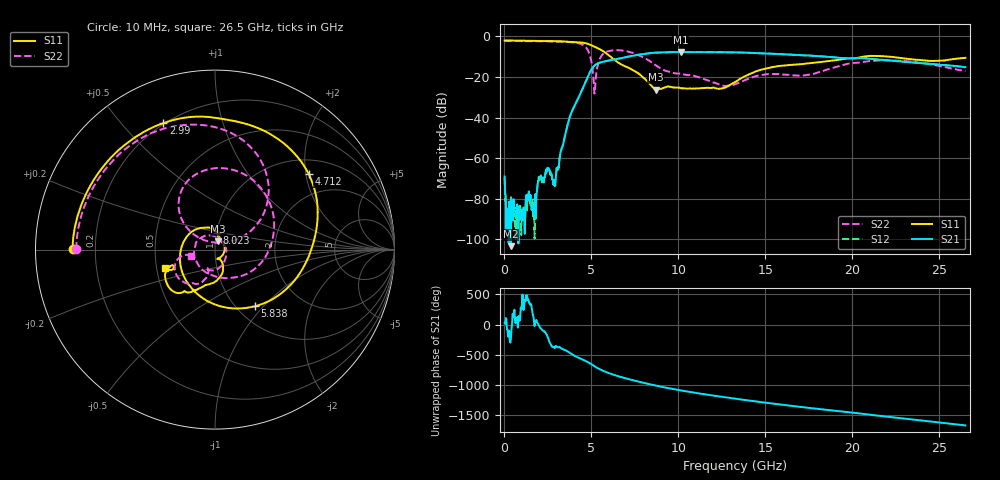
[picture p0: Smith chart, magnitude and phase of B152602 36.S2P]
!  2-Port S-parameters saved by WinCal
! VAR MeasName=S-Parameters (CALIBRATED_DATA) read from VNA (N5242A)
! VAR MeasDate=2016-1-5 16:31:28
! VAR NAME=B152602 36
! VAR FILENAME=B152602 36.S2P
! VAR DATE=2016-1-5 16:31:28
! VAR PHYS_PORTS=1,2
# Hz S DB R 50
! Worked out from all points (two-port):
!   801 points, 10 MHz to 26.5 GHz, reference 50 ohm
!   highest |S21| = -7.67 dB at 10.14 GHz (marker M1); lowest = -103.3 dB at 374.2 MHz (marker M2)
!   |S21| within 3 dB of the highest: 6.748 GHz to 19.42 GHz (12.67 GHz wide, 96.8 % of centre); 20.43028 GHz to 20.45867 GHz (28.39 MHz wide, 0.139 % of centre)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
!   lowest |S11| = -26.2 dB at 8.685 GHz (marker M3), VSWR 1.10, Z = 51.6 + j4.71 ohm
!   |S11| at or under -10 dB: 6.094 GHz to 20.61 GHz (14.51 GHz wide, 109 % of centre); 22.15 GHz to end of sweep
!   |S22| runs from -28.1 to -2.2 dB; largest |S21 - S12| = 0.0032
!   S11 on the Smith chart (normalised r, x): 10 MHz: 0.12, +0.00; 2.99 GHz: 0.20, +0.65; 4.712 GHz: 1.35, +2.07; 5.838 GHz: 1.21, -0.90; 8.023 GHz: 1.01, +0.19; 26.5 GHz: 0.55, -0.12
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1e7  -2.01 179.7  -68.96 24.1  -69.51 1.8  -2.24 179.8
3.742375e8  -2.04 172.2  -103.30 139.0  -79.12 179.1  -2.25 174.2
1.698738e9  -2.20 144.7  -85.25 56.7  -81.88 65.4  -2.36 153.3
2.460325e9  -2.29 126.8  -65.82 176.2  -64.70 172.4  -2.44 139.9
2.990125e9  -2.37 112.2  -64.90 -1.7  -66.91 -6.5  -2.51 129.0
3.7186e9  -2.72 88.0  -40.82 -101.0  -40.80 -101.2  -2.78 109.8
4.447075e9  -3.06 55.4  -26.71 147.5  -26.72 147.7  -3.89 77.9
4.711975e9  -3.46 39.0  -21.41 111.7  -21.43 111.8  -5.68 57.2
5.17555e9  -5.07 6.4  -14.40 30.2  -14.40 30.3  -28.15 76.0
5.8378e9  -8.25 -54.7  -12.18 -65.4  -12.16 -65.3  -7.72 111.9
6.6325e9  -13.42 -153.6  -10.88 -142.4  -10.88 -142.3  -6.86 74.2
8.023225e9  -20.54 82.3  -8.69 113.7  -8.68 113.8  -10.52 -1.3
8.685475e9  -26.21 68.7  -8.05 70.5  -8.04 70.5  -14.15 -51.2
8.851038e9  -25.97 70.5  -7.98 60.6  -7.97 60.5  -15.10 -64.6
1.014242e10  -25.47 -6.8  -7.67 -10.2  -7.67 -10.2  -18.44 -168.1
1.16656e10  -25.28 -69.2  -7.76 -80.9  -7.75 -80.8  -21.61 107.0
1.3255e10  -22.49 -60.7  -7.89 -146.3  -7.89 -146.3  -23.60 -17.4
1.567221e10  -14.72 -91.9  -8.67 123.5  -8.66 123.4  -18.49 -109.3
1.769208e10  -13.08 -109.3  -9.54 54.4  -9.50 54.5  -18.59 -108.5
2.007618e10  -10.84 -126.6  -10.74 -19.8  -10.74 -19.8  -13.09 -120.9
2.209604e10  -9.96 -150.9  -11.84 -87.2  -11.79 -87.6  -11.79 -145.1
2.65e10  -10.56 -159.8  -15.17 130.2  -15.16 130.1  -17.09 -164.9
